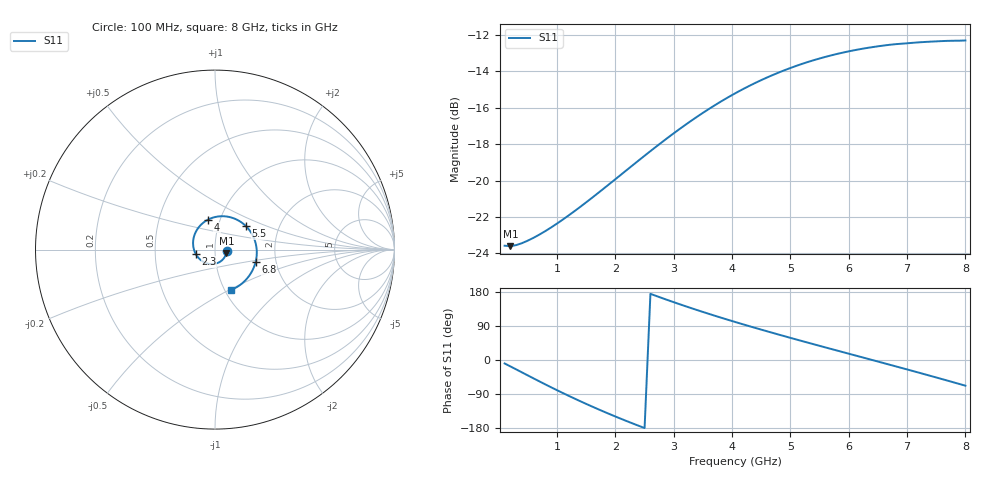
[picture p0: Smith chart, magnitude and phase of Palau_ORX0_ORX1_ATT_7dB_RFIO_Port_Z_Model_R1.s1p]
! Created Fri Oct  9 14:29:22 2020
! Palau ORX0/ORX1 RFIO Port Impedance Model.
! Attenuation  : 7 dB.
! Revision		: R1.
! Impedance Mode 	: Balanced Differential-Mode.
! Impedance Format 	: Series Equivalent Differential Impedance (SEDZ).
# hz S ma R 100
! 1 Port Network Data from SP1.SP block
! freq  magS11  angS11
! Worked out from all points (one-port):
!   80 points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, 100 MHz to 8 GHz, reference 100 ohm
!   lowest |S11| = -23.6 dB at 200 MHz (marker M1), VSWR 1.14, Z = 113 - j4.4 ohm
!   |S11| at or under -10 dB: start of sweep to end of sweep
!   S11 on the Smith chart (normalised r, x): 100 MHz: 1.14, -0.02; 2.3 GHz: 0.80, -0.04; 4 GHz: 0.88, +0.30; 5.5 GHz: 1.36, +0.37; 6.8 GHz: 1.57, -0.22; 8 GHz: 1.08, -0.51
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1e8  0.06626 -9.1
2e8  0.06608 -17.0
4e8  0.06737 -32.9
6e8  0.06972 -48.8
1.1e9  0.07821 -87.3
1.4e9  0.08478 -109.0
1.6e9  0.08972 -122.8
1.8e9  0.0951 -136.2
2.1e9  0.1039 -155.4
2.3e9  0.1103 -167.7
2.7e9  0.124 169.0
3.1e9  0.1385 147.2
3.5e9  0.1534 126.8
4e9  0.1716 102.8
4.1e9  0.1752 98.2
4.4e9  0.1854 84.6
4.6e9  0.1918 75.7
4.8e9  0.1979 67.0
5.1e9  0.2063 54.2
5.5e9  0.2162 37.4
5.8e9  0.2225 24.9
6.1e9  0.2279 12.5
6.5e9  0.2335 -4.1
6.8e9  0.2367 -16.6
7.1e9  0.2387 -29.1
7.5e9  0.2409 -46.1
7.7e9  0.2417 -54.7
8e9  0.2423 -67.8
